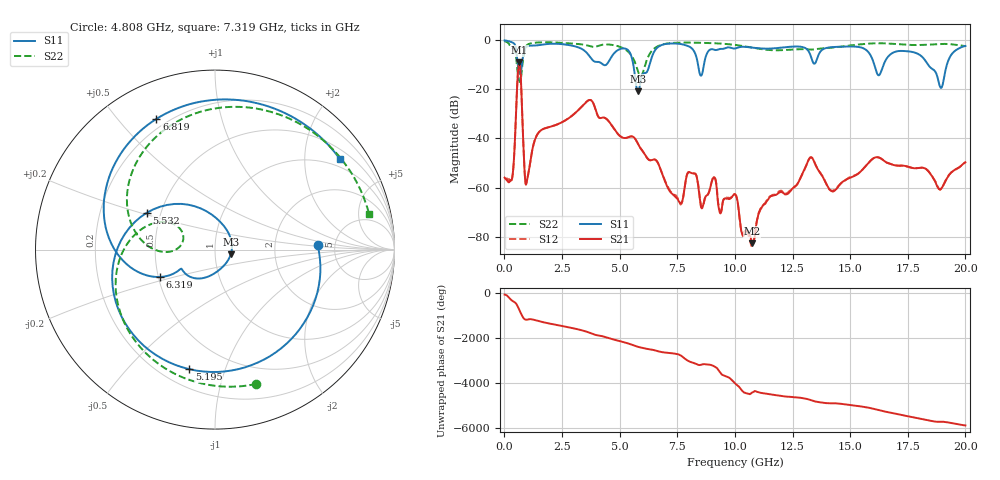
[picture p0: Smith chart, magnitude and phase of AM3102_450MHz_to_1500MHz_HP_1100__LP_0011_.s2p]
!Agilent Technologies,E8364B,MY43040894,A.07.50.67
!Agilent E8364B: A.07.50.67
!Date: Thursday, January 11, 2018 06:32:38
!Correction: S11(Full 2 Port(1,2))
!S21(Full 2 Port(1,2))
!S12(Full 2 Port(1,2))
!S22(Full 2 Port(1,2))
!S2P File: Measurements: S11, S21, S12, S22:
# Hz S  dB  R 50
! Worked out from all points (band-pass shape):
!   1601 points, 10 MHz to 20 GHz, reference 50 ohm
!   highest |S21| = -9.00 dB at 647.2 MHz (marker M1); lowest = -82.7 dB at 10.74 GHz (marker M2)
!   |S21| within 3 dB of the highest: 597.8 MHz to 694.8 MHz (97.02 MHz wide, 15 % of centre)
!   lowest |S11| = -20.8 dB at 5.795 GHz (marker M3), VSWR 1.20, Z = 59.6 - j3.08 ohm
!   |S11| at or under -10 dB: 5.594 GHz to 6.299 GHz (704.3 MHz wide, 11.8 % of centre); 16.05 GHz to 16.45 GHz (399.8 MHz wide, 2.46 % of centre); 18.38 GHz to 19.2 GHz (811.8 MHz wide, 4.32 % of centre)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
!   |S22| runs from -17.0 to -0.4 dB; largest |S21 - S12| = 0.0017
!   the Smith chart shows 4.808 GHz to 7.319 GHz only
!   S11 on the Smith chart (normalised r, x): 4.808 GHz: 3.66, +0.27; 5.195 GHz: 0.31, -0.76; 5.532 GHz: 0.42, +0.21; 6.319 GHz: 0.51, -0.18; 6.819 GHz: 0.16, +0.64; 7.319 GHz: 0.76, +2.92
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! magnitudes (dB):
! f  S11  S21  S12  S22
! 10 MHz  -0.1  -56.0  -56.7  -0.4
! 334.8 MHz  -0.9  -56.2  -56.4  -3.2
! 647.2 MHz  -13.2  -9.0  -9.0  -16.6
! 972 MHz  -2.6  -57.4  -57.4  -2.1
! 1.484 GHz  -2.0  -37.6  -37.6  -0.9
! 3.346 GHz  -3.5  -27.1  -27.1  -1.7
! 4.808 GHz  -4.8  -36.7  -36.8  -2.1
! 5.195 GHz  -3.3  -39.8  -39.8  -3.5
! 5.532 GHz  -7.3  -39.1  -39.2  -6.5
! 5.795 GHz  -20.8  -42.1  -42.2  -12.6
! 6.319 GHz  -9.3  -48.9  -48.9  -5.3
! 6.682 GHz  -2.7  -50.4  -50.4  -2.3
! 6.819 GHz  -2.0  -53.7  -53.7  -1.8
! 7.319 GHz  -1.3  -62.9  -62.7  -1.1
! 8.531 GHz  -14.4  -67.8  -67.3  -1.0
! 10.01 GHz  -3.4  -62.7  -62.7  -1.9
! 10.74 GHz  -3.0  -82.7  -83.8  -3.0
! 13.34 GHz  -7.8  -47.8  -47.8  -3.8
! 14.24 GHz  -2.8  -61.6  -61.3  -3.0
! 16.68 GHz  -6.4  -50.2  -50.2  -1.3
! 18.94 GHz  -19.4  -60.5  -60.6  -1.5
! 20 GHz  -2.3  -49.7  -49.8  -2.4
